| TEXAS INSTRUMENTS INCORPORATED
| Standard Linear and Logic Group
| IBIS Model of SN74CBT3251
| 1-OF-8 FET MULTIPLEXER/DEMULTIPLEXER
| This file contains package information for the following:
|  SOIC 16-pin (D) package as [Component] CBT3251_D
|  SSOP 16-pin (DB) package as [Component] CBT3251_DB
|  SSOP 16-pin (DBQR) package as [Component] CBT3251_DBQ
|  TSSOP 16-pin (PW) package as [Component] CBT3251_PW
|  QFN 16-pin (RGY) package as [Component] CBT3251_RGY
| This device can be powered at the following Vccs:
|  5 volt Vcc
|  4 volt Vcc
| This file provides unique models under the [Model Selector] for each Vcc.
| For operation at a specific Vcc, select the appropriate model after each
| [Model Selector] keyword.
[IBIS Ver]   3.2
[Comment char]  |_char
[File Name]   sn74cbt3251.ibs
[File Rev]   1.1 | a_die
[Date]   May 27, 2003
[Source]   Data created from TI-SPICE simulations at TI-SLL.
[Notes]   The following is an IBIS list for the CBT3251.
   Please contact sllibis@ti.com with questions and
   comments concerning SLL IBIS models.
   This IBIS model is created from a BA (back annotated
   netlist).
   - Power-clamp data has been deleted since there is no
   power-clamp diode in the device.
   - Non-monotonic data due to FET characteristics.
[Disclaimer] Property of Texas Instruments Incorporated.  Unauthorized
   reproduction and/or distribution is strictly prohibited.
   This product is protected under copyright law.
   Created  2003, (C) Copyright  2003, Texas Instruments
   Incorporated, All Rights Reserved
   UNLESS THERE IS A SIGNED, WRITTEN AGREEMENT TO THE
   CONTRARY, TEXAS INSTRUMENTS (TI) IS PROVIDING THE IBIS
   MODELS  AND WITHOUT ANY WARRANTY, EXPRESSED OR
   IMPLIED.  TI assumes no liability for:
   1) the accuracy of the IBIS models provided to your
   company;
   2) the proper functioning of these IBIS Models in your
   design or for any resulting applications; or
   3) infringement of patents, copyrights or intellectual
   property rights resulting from your use of these IBIS
   models.
   TI provides IBIS Models as a service to our customers.
   You and your company shall not distribute, sell or give
   these models to anyone else without prior written
   permission from TI.
   TI reserves the right to make changes to our products or
   to discontinue any semiconductor product or service
   without notice, and advises our customers to obtain the
   latest version of relevant information to verify, before
   placing orders, that the information being relied on is
   current.
   Please be aware that your receipt and use of the IBIS
   information provided shall serve as acceptance of these
   terms and conditions.  If you do not accept these terms,
   you should return or destroy the IBIS models and any
   other accompanying information immediately.
| Component CBT3251_D 16-pin SOIC
[Component]   CBT3251_D
[Manufacturer]   Texas Instruments, Inc.
[Package]
|   typ   min   max
R_pkg   3.900e-02   2.800e-02   4.900e-02
L_pkg   3.453e-09   2.350e-09   4.375e-09
C_pkg   5.210e-13   2.540e-13   7.080e-13
[Pin]   signal_name   model_name   R_pin   L_pin   C_pin
1   B4   CBT3251_IO   4.200e-02   4.336e-09   7.030e-13
2   B3   CBT3251_IO   4.900e-02   3.778e-09   6.340e-13
3   B2   CBT3251_IO   2.800e-02   3.449e-09   5.180e-13
4   B1   CBT3251_IO   2.900e-02   2.393e-09   2.540e-13
5   A   CBT3251_IO   2.800e-02   2.350e-09   2.640e-13
6   NC   NC   4.800e-02   3.312e-09   4.830e-13
7   NOE   CBT3251_OE   4.300e-02   3.629e-09   6.040e-13
8   GND   GND   4.400e-02   4.375e-09   7.080e-13
9   S2   CBT3251_SEL   4.200e-02   4.336e-09   7.030e-13
10   S1   CBT3251_SEL   4.900e-02   3.778e-09   6.340e-13
11   S0   CBT3251_SEL   2.800e-02   3.449e-09   5.180e-13
12   B8   CBT3251_IO   2.900e-02   2.393e-09   2.550e-13
13   B7   CBT3251_IO   2.800e-02   2.350e-09   2.640e-13
14   B6   CBT3251_IO   4.800e-02   3.312e-09   4.830e-13
15   B5   CBT3251_IO   4.300e-02   3.629e-09   6.040e-13
16   VCC   POWER   4.400e-02   4.375e-09   7.080e-13
| Component CBT3251_DB 16-pin SSOP
[Component]   CBT3251_DB
[Manufacturer]   Texas Instruments, Inc.
[Package]
|   typ   min   max
R_pkg   4.800e-02   4.600e-02   5.000e-02
L_pkg   3.536e-09   3.213e-09   3.798e-09
C_pkg   3.760e-13   3.140e-13   4.400e-13
[Pin]   signal_name   model_name   R_pin   L_pin   C_pin
1   B4   CBT3251_IO   4.800e-02   3.797e-09   3.770e-13
2   B3   CBT3251_IO   4.600e-02   3.723e-09   4.400e-13
3   B2   CBT3251_IO   4.800e-02   3.409e-09   3.720e-13
4   B1   CBT3251_IO   4.900e-02   3.213e-09   3.140e-13
5   A   CBT3251_IO   4.900e-02   3.213e-09   3.140e-13
6   NC   NC   4.800e-02   3.409e-09   3.720e-13
7   NOE   CBT3251_OE   4.600e-02   3.723e-09   4.400e-13
8   GND   GND   4.800e-02   3.798e-09   3.770e-13
9   S2   CBT3251_SEL   4.800e-02   3.797e-09   3.770e-13
10   S1   CBT3251_SEL   4.600e-02   3.725e-09   4.400e-13
11   S0   CBT3251_SEL   4.800e-02   3.409e-09   3.720e-13
12   B8   CBT3251_IO   4.900e-02   3.214e-09   3.140e-13
13   B7   CBT3251_IO   5.000e-02   3.216e-09   3.140e-13
14   B6   CBT3251_IO   4.800e-02   3.409e-09   3.720e-13
15   B5   CBT3251_IO   4.700e-02   3.729e-09   4.400e-13
16   VCC   POWER   4.800e-02   3.797e-09   3.770e-13
| Component CBT3251_DBQ 16-pin SSOP
[Component]   CBT3251_DBQ
[Manufacturer]   Texas Instruments, Inc.
[Package]
|   typ   min   max
R_pkg   3.800e-02   2.700e-02   5.900e-02
L_pkg   2.353e-09   1.491e-09   4.500e-09
C_pkg   2.100e-13   6.400e-14   5.920e-13
[Pin]   signal_name   model_name   R_pin   L_pin   C_pin
1   B4   CBT3251_IO   5.800e-02   4.450e-09   5.920e-13
2   B3   CBT3251_IO   4.000e-02   1.930e-09   1.110e-13
3   B2   CBT3251_IO   2.800e-02   1.538e-09   7.600e-14
4   B1   CBT3251_IO   2.700e-02   1.491e-09   6.400e-14
5   A   CBT3251_IO   2.700e-02   1.491e-09   6.400e-14
6   NC   NC   2.700e-02   1.506e-09   7.500e-14
7   NOE   CBT3251_OE   3.300e-02   1.922e-09   1.090e-13
8   GND   GND   5.900e-02   4.500e-09   5.880e-13
9   S2   CBT3251_SEL   5.800e-02   3.695e-09   4.140e-13
10   S1   CBT3251_SEL   3.400e-02   2.685e-09   2.820e-13
11   S0   CBT3251_SEL   2.900e-02   1.552e-09   7.700e-14
12   B8   CBT3251_IO   2.800e-02   1.506e-09   6.500e-14
13   B7   CBT3251_IO   2.700e-02   1.492e-09   6.400e-14
14   B6   CBT3251_IO   2.800e-02   1.534e-09   7.600e-14
15   B5   CBT3251_IO   4.000e-02   2.703e-09   2.840e-13
16   VCC   POWER   5.600e-02   3.645e-09   4.180e-13
| Component CBT3251_PW 16-pin TSSOP
[Component]   CBT3251_PW
[Manufacturer]   Texas Instruments, Inc.
[Package]
|   typ   min   max
R_pkg   4.500e-02   3.800e-02   5.100e-02
L_pkg   2.593e-09   2.447e-09   3.080e-09
C_pkg   2.810e-13   2.430e-13   3.770e-13
[Pin]   signal_name   model_name   R_pin   L_pin   C_pin
1   B4   CBT3251_IO   4.000e-02   3.080e-09   3.770e-13
2   B3   CBT3251_IO   3.800e-02   2.458e-09   2.810e-13
3   B2   CBT3251_IO   5.100e-02   2.512e-09   2.550e-13
4   B1   CBT3251_IO   5.100e-02   2.447e-09   2.430e-13
5   A   CBT3251_IO   5.100e-02   2.447e-09   2.430e-13
6   NC   NC   5.100e-02   2.512e-09   2.550e-13
7   NOE   CBT3251_OE   3.800e-02   2.458e-09   2.810e-13
8   GND   GND   4.000e-02   3.080e-09   3.770e-13
9   S2   CBT3251_SEL   3.900e-02   2.832e-09   3.160e-13
10   S1   CBT3251_SEL   3.800e-02   2.460e-09   2.790e-13
11   S0   CBT3251_SEL   5.100e-02   2.512e-09   2.550e-13
12   B8   CBT3251_IO   5.100e-02   2.447e-09   2.430e-13
13   B7   CBT3251_IO   5.100e-02   2.447e-09   2.430e-13
14   B6   CBT3251_IO   5.100e-02   2.512e-09   2.550e-13
15   B5   CBT3251_IO   3.800e-02   2.459e-09   2.790e-13
16   VCC   POWER   3.900e-02   2.832e-09   3.160e-13
| Component CBT3251_RGY 16-pin QFN
[Component]   CBT3251_RGY
[Manufacturer]   Texas Instruments, Inc.
[Package]
|   typ   min   max
R_pkg   3.000e-02   2.700e-02   3.800e-02
L_pkg   8.000e-10   7.220e-10   9.400e-10
C_pkg   1.410e-13   1.290e-13   1.550e-13
[Pin]   signal_name   model_name   R_pin   L_pin   C_pin
1   B4   CBT3251_IO   2.700e-02   8.180e-10   1.320e-13
2   B3   CBT3251_IO   2.700e-02   8.030e-10   1.300e-13
3   B2   CBT3251_IO   3.700e-02   9.080e-10   1.500e-13
4   B1   CBT3251_IO   2.900e-02   7.220e-10   1.390e-13
5   A   CBT3251_IO   2.900e-02   7.220e-10   1.390e-13
6   NC   NC   2.900e-02   7.300e-10   1.400e-13
7   NOE   CBT3251_OE   2.900e-02   7.240e-10   1.390e-13
8   GND   GND   3.100e-02   8.000e-10   1.400e-13
9   S2   CBT3251_SEL   2.700e-02   8.110e-10   1.290e-13
10   S1   CBT3251_SEL   2.800e-02   7.840e-10   1.310e-13
11   S0   CBT3251_SEL   3.700e-02   9.150e-10   1.530e-13
12   B8   CBT3251_IO   2.900e-02   8.470e-10   1.520e-13
13   B7   CBT3251_IO   2.900e-02   7.580e-10   1.430e-13
14   B6   CBT3251_IO   2.900e-02   7.720e-10   1.440e-13
15   B5   CBT3251_IO   2.900e-02   7.400e-10   1.420e-13
16   VCC   POWER   3.800e-02   9.400e-10   1.550e-13
[Series Switch Groups]
| Function Group States
On  1 /   | A->B1 OE\ LOW S2-S0 LOW
On  2 /   | A->B2 OE\ LOW S2-S1 LOW SO HIGH
On  3 /   | A->B3 OE\ LOW S2,S2 LOW S1 HIGH
On  4 /   | A->B4 OE\ LOW S2 LOW S1-S0 HIGH
On  5 /   | A->B5 OE\ LOW S2 HIGH S1-S0 LOW
On  6 /   | A->B6 OE\ LOW S2,S0 HIGH S1 LOW
On  7 /   | A->B7 OE\ LOW S2-S1 HIGH S0 LOW
On  8 /   | A->B8 OE\ LOW S2-S0 HIGH
[Series Pin Mapping]   pin_2   model_name   function_table_group
5   4   CBT3251_IO_50_S   1
| 5   4   CBT3251_IO_40_S   1
5   3   CBT3251_IO_50_S   2
| 5   3   CBT3251_IO_40_S   2
5   2   CBT3251_IO_50_S   3
| 5   2   CBT3251_IO_40_S   3
5   1   CBT3251_IO_50_S   4
| 5   1   CBT3251_IO_40_S   4
5   15   CBT3251_IO_50_S   5
| 5   15   CBT3251_IO_40_S   5
5   14   CBT3251_IO_50_S   6
| 5   14   CBT3251_IO_40_S   6
5   13   CBT3251_IO_50_S   7
| 5   13   CBT3251_IO_40_S   7
5   12   CBT3251_IO_50_S   8
| 5   12   CBT3251_IO_40_S   8
| Model CBT3251_OE
[Model Selector]   CBT3251_OE
CBT3251_OE_50   5 volt Vcc
CBT3251_OE_40   4 volt Vcc
| Model CBT3251_SEL
[Model Selector]   CBT3251_SEL
CBT3251_SEL_50   5 volt Vcc
CBT3251_SEL_40   4 volt Vcc
| Model CBT3251_IO
[Model Selector]   CBT3251_IO
CBT3251_IO_50   5 volt Vcc
CBT3251_IO_40   4 volt Vcc
| Model CBT3251_IO_S
[Model Selector]   CBT3251_IO_S
CBT3251_IO_50_S   5 volt Vcc
CBT3251_IO_40_S   4 volt Vcc
[Model]   CBT3251_IO_50_S
Model_type  Series_switch
| variable   typ   min   max
C_comp   0   0   0
[Temperature Range]   40   100   -40
| Ambient temperature   25   85   -40
[Voltage range]   5   4.5   5.5
[On]
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[Off]
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[Model]   CBT3251_IO_40_S
Model_type  Series_switch
| variable   typ   min   max
C_comp   0   0   0
[Temperature Range]   40   100   -40
| Ambient temperature   25   85   -40
[Voltage range]   4   4   4
[On]
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[Off]
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| Models and submodels in the file (8): CBT3251_OE_50 (Input), CBT3251_OE_40 (Input), CBT3251_SEL_50 (Input), CBT3251_SEL_40 (Input), CBT3251_IO_50_S (Series_switch), CBT3251_IO_50 (Terminator), CBT3251_IO_40_S (Series_switch), CBT3251_IO_40 (Terminator)
